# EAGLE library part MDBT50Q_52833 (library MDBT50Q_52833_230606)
Raytac Corporation Part Number: MDBT50Q-512K / MDBT50Q-P512K / MDBT50Q-U512K Bluetooth Low Energy Module based on Noridc nRF52833 Size: 15.5x10.5mm Source: Raytac datasheet
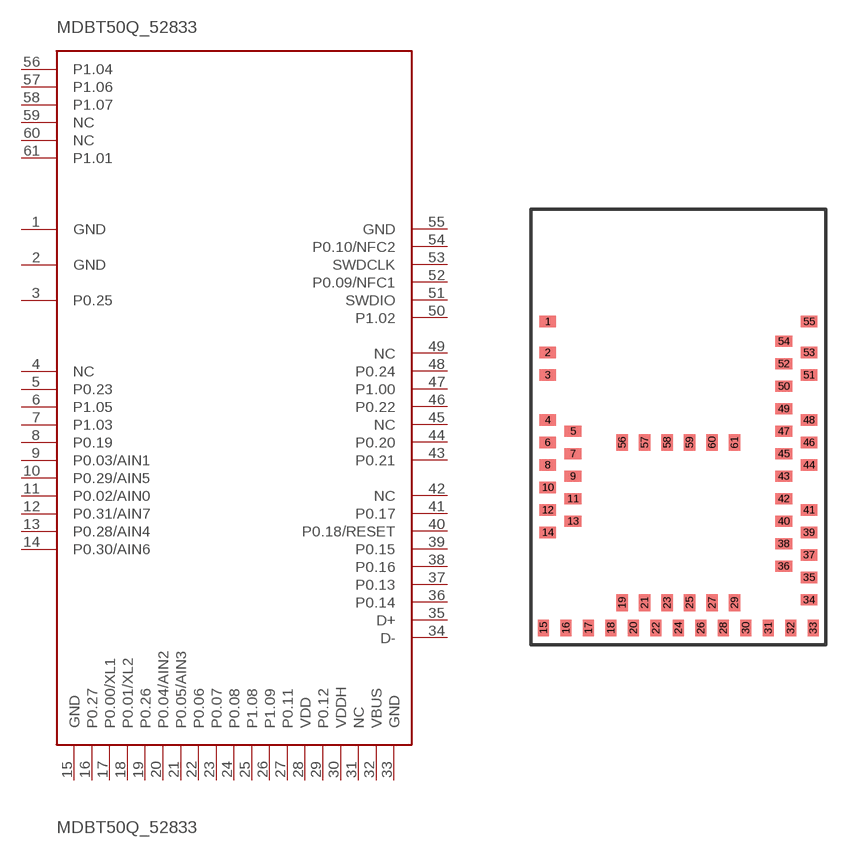
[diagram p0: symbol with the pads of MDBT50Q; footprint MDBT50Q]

Designator prefix MDBT50Q_52833

## MDBT50Q_52833  [MDBT50Q]
1  GND
2  GND
3  P0.25
4  NC
5  P0.23
6  P1.05
7  P1.03
8  P0.19
9  P0.03/AIN1
10  P0.29/AIN5
11  P0.02/AIN0
12  P0.31/AIN7
13  P0.28/AIN4
14  P0.30/AIN6
15  GND
16  P0.27
17  P0.00/XL1
18  P0.01/XL2
19  P0.26
20  P0.04/AIN2
21  P0.05/AIN3
22  P0.06
23  P0.07
24  P0.08
25  P1.08
26  P1.09
27  P0.11
28  VDD
29  P0.12
30  VDDH
31  NC
32  VBUS
33  GND
34  D-
35  D+
36  P0.14
37  P0.13
38  P0.16
39  P0.15
40  P0.18/RESET
41  P0.17
42  NC
43  P0.21
44  P0.20
45  NC
46  P0.22
47  P1.00
48  P0.24
49  NC
50  P1.02
51  SWDIO
52  P0.09/NFC1
53  SWDCLK
54  P0.10/NFC2
55  GND
56  P1.04
57  P1.06
58  P1.07
59  NC
60  NC
61  P1.01

## Footprint MDBT50Q (pad centres in mm)
Raytac Corporation Part Number: MDBT50Q-1MV2 / MDBT50Q-P1MV2 MDBT50Q-512K / MDBT50Q-P512K Bluetooth Low Energy Module based on Noridc nRF52840 / nRF52833 Size: 15.5x10.5mm Source: Raytac datasheet
smd 0.6 x 0.4: 1 -4.65,3.75; 2 -4.65,2.65; 3 -4.65,1.85; 4 -4.65,0.25; 5 -3.75,-0.15; 6 -4.65,-0.55; 7 -3.75,-0.95; 8 -4.65,-1.35; 9 -3.75,-1.75; 10 -4.65,-2.15; 11 -3.75,-2.55; 12 -4.65,-2.95; 13 -3.75,-3.35; 14 -4.65,-3.75; 34 4.65,-6.15; 35 4.65,-5.35; 36 3.75,-4.95; 37 4.65,-4.55; 38 3.75,-4.15; 39 4.65,-3.75; 40 3.75,-3.35; 41 4.65,-2.95; 42 3.75,-2.55; 43 3.75,-1.75; 44 4.65,-1.35; 45 3.75,-0.95; 46 4.65,-0.55; 47 3.75,-0.15; 48 4.65,0.25; 49 3.75,0.65; 50 3.75,1.45; 51 4.65,1.85; 52 3.75,2.25; 53 4.65,2.65; 54 3.75,3.05; 55 4.65,3.75
smd 0.4 x 0.6: 15 -4.8,-7.15; 16 -4,-7.15; 17 -3.2,-7.15; 18 -2.4,-7.15; 19 -2,-6.25; 20 -1.6,-7.15; 21 -1.2,-6.25; 22 -0.8,-7.15; 23 -0.4,-6.25; 24 0,-7.15; 25 0.4,-6.25; 26 0.8,-7.15; 27 1.2,-6.25; 28 1.6,-7.15; 29 2,-6.25; 30 2.4,-7.15; 31 3.2,-7.15; 32 4,-7.15; 33 4.8,-7.15; 56 -2,-0.55; 57 -1.2,-0.55; 58 -0.4,-0.55; 59 0.4,-0.55; 60 1.2,-0.55; 61 2,-0.55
